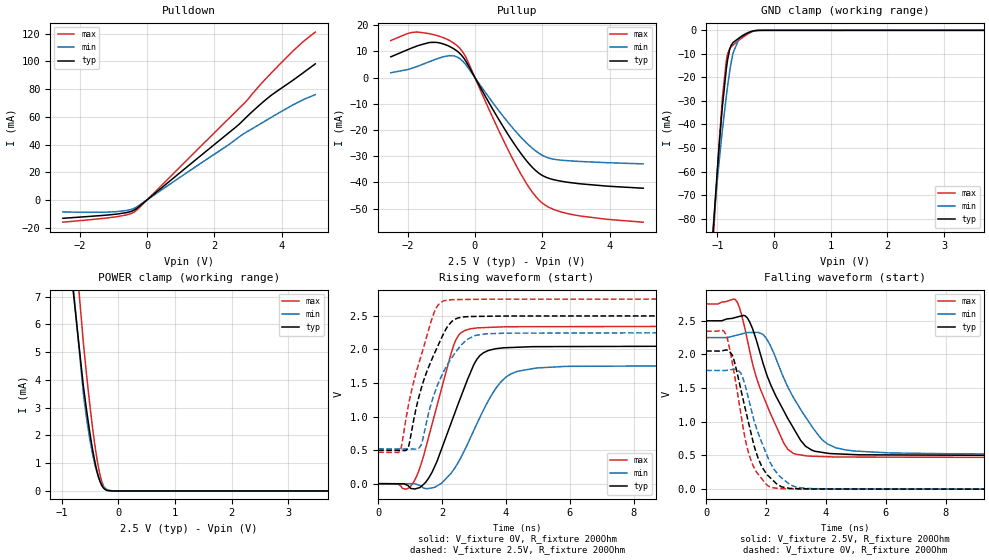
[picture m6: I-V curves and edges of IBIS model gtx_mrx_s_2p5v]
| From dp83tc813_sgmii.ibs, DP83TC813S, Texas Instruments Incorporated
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| gtx_mrx_s_2p5v
[Model]   gtx_mrx_s_2p5v
Model_type   I/O
Polarity   Non-Inverting
Enable   Active-Low
Vinl = 0.7
Vinh = 1.7
Vmeas = 1.25
Vref = 1.25
Cref = 2pF
Rref = 100000
|   typ   min   max
C_comp   2.76pF   2.73pF   2.77pF
[Voltage Range]   2.5   2.25   2.75
[Temperature Range]   27   150   -40
[Pullup Reference]   2.5   2.25   2.75
[Pulldown Reference]   0   0   0
[Power Clamp Reference]   2.5   2.25   2.75
[GND Clamp Reference]   0   0   0
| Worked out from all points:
|   slope of the pulldown table from 0 to 0.375 V, typ, clamps not added: 49.7 ohm
|   slope of the pullup table from 0 to 0.375 V, typ, clamps not added: 43.5 ohm
|   GND clamp passes 1 mA (typ) near -0.45 V on its own axis
|   POWER clamp passes 1 mA (typ) near -0.41 V on its own axis
|   falling waveform, V_fixture 2.5V, R_fixture 200Ohm: 20-80 % time 1.18ns typ, 1.28ns min, 1.01ns max; typ from 2.5 V to 0.498 V
|   rising waveform, V_fixture 0V, R_fixture 200Ohm: 20-80 % time 975ps typ, 1.12ns min, 794ps max; typ from 0 V to 2.05 V
|   rising waveform, V_fixture 2.5V, R_fixture 200Ohm: 20-80 % time 823ps typ, 856ps min, 727ps max; typ from 0.498 V to 2.5 V
|   falling waveform, V_fixture 0V, R_fixture 200Ohm: 20-80 % time 706ps typ, 814ps min, 592ps max; typ from 2.05 V to 0 V
[Pulldown]
|   Voltage   I(typ)   I(min)   I(max)
-2.5V     -13.29mA   -8.687mA   -16.1mA
-925mV    -10.31mA   -8.492mA   -12.22mA
-512.5mV  -8.603mA   -7.139mA   -10.18mA
-347.5mV  -6.835mA   -5.631mA   -8.211mA
2.638V    52.57mA    43.69mA    63.75mA
2.885V    58.13mA    47.96mA    69.7mA
3.462V    71.02mA    56.29mA    85.76mA
3.958V    80.11mA    63.41mA    98.27mA
4.633V    91.66mA    72.28mA    114.2mA
5V        98.27mA    76.01mA    121.2mA
[GND Clamp]
|   Voltage   I(typ)   I(min)   I(max)
-2.5V     -649.6mA   -557.1mA   -724.7mA
-1.097V   -92.84mA   -90.08mA   -98.6mA
-1.03V    -68.96mA   -71.19mA   -71.1mA
-962.5mV  -46.84mA   -53.94mA   -45.4mA
-917.5mV  -33.74mA   -43.48mA   -30.33mA
-835mV    -14.88mA   -26.4mA    -11.64mA
-782.5mV  -7.979mA   -17.25mA   -7.714mA
-722.5mV  -5.135mA   -9.451mA   -6.216mA
-617.5mV  -3.252mA   -3.474mA   -4.173mA
-497.5mV  -1.53mA    -1.353mA   -2.064mA
-265mV    -14.91uA   -36.81uA   -15.25uA
5V        0A         0A         0A
[Pullup]
|   Voltage   I(typ)   I(min)   I(max)
-2.5V     7.944mA    1.866mA    14.16mA
-1.847V   11.46mA    3.684mA    17.29mA
-1.315V   13.45mA    6.279mA    16.67mA
-752.5mV  11.89mA    8.383mA    14.16mA
-460mV    9.358mA    7.341mA    11.34mA
-257.5mV  5.988mA    4.704mA    7.488mA
642.5mV   -14.55mA   -11.48mA   -18.41mA
1.272V    -27.27mA   -21.43mA   -34.67mA
1.677V    -33.87mA   -26.64mA   -43.23mA
2.007V    -37.38mA   -29.68mA   -47.92mA
2.953V    -40.27mA   -31.87mA   -52.42mA
5V        -42.22mA   -32.93mA   -55.18mA
[POWER Clamp]
|   Voltage   I(typ)   I(min)   I(max)
-2.5V     111.4mA    76.2mA     154.9mA
-1.06V    12.26mA    13.09mA    16.05mA
-617.5mV  3.803mA    3.523mA    5.367mA
-557.5mV  2.879mA    2.591mA    4.147mA
-505mV    2.141mA    1.896mA    3.157mA
-445mV    1.398mA    1.242mA    2.137mA
-392.5mV  857.5uA    791.8uA    1.369mA
-347.5mV  495.5uA    495.4uA    828.3uA
-302.5mV  241.6uA    280.7uA    419.5uA
-220mV    36.63uA    73.03uA    55.79uA
-2.5mV    0A         70.01nA    0A
5V        0A         0A         0A
[Ramp]
R_load = 200
|   typ   min   max
dV/dt_r   1.23037/9.67486e-10   1.05666/1.12067e-09   1.40715/7.92973e-10
dV/dt_f   1.20096/1.16812e-09   1.03799/1.27155e-09   1.36848/1.00485e-09
[Falling Waveform]
V_fixture = 2.5V
V_fixture_min = 2.25V
V_fixture_max = 2.75V
R_fixture = 200Ohm
C_fixture = 0F
|   Time   V(typ)   V(min)   V(max)
0s        2.5V       2.25V      2.75V
1.029ns   2.555V     2.286V     2.785V
1.454ns   2.484V     2.325V     2.054V
1.924ns   1.839V     2.285V     1.366V
2.596ns   1.161V     1.649V     682.7mV
2.901ns   919.2mV    1.374V     534.6mV
3.324ns   636.6mV    1.07V      496.4mV
3.877ns   545.8mV    734.2mV    484.4mV
4.637ns   519.3mV    584.3mV    477.1mV
12ns      498.4mV    519.9mV    469.2mV
[Rising Waveform]
V_fixture = 0V
V_fixture_min = 0V
V_fixture_max = 0V
R_fixture = 200Ohm
C_fixture = 0F
|   Time   V(typ)   V(min)   V(max)
0s        25.62uV    133.3uV    11.85uV
855.4ps   -12.29mV   -959.5uV   -81.82mV
1.125ns   -77.92mV   -1.304mV   36.02mV
1.693ns   175mV      -62.08mV   895.2mV
2.363ns   1.004V     207.9mV    2.057V
2.722ns   1.456V     513.7mV    2.283V
3.298ns   1.95V      1.097V     2.325V
3.836ns   2.019V     1.511V     2.334V
4.377ns   2.032V     1.675V     2.338V
12ns      2.051V     1.761V     2.345V
[Rising Waveform]
V_fixture = 2.5V
V_fixture_min = 2.25V
V_fixture_max = 2.75V
R_fixture = 200Ohm
C_fixture = 0F
|   Time   V(typ)   V(min)   V(max)
0s        498.4mV    519.9mV    469.2mV
704.5ps   494.1mV    517mV      505.9mV
933.8ps   533.5mV    516mV      1.137V
1.347ns   1.416V     577.2mV    1.91V
1.762ns   1.94V      1.342V     2.561V
2.039ns   2.225V     1.66V      2.72V
2.314ns   2.42V      1.882V     2.74V
2.794ns   2.488V     2.149V     2.744V
3.401ns   2.494V     2.233V     2.748V
12ns      2.5V       2.25V      2.75V
[Falling Waveform]
|Gnd
V_fixture = 0V
V_fixture_min = 0V
V_fixture_max = 0V
R_fixture = 200Ohm
C_fixture = 0F
|   Time   V(typ)   V(min)   V(max)
0s        2.052V     1.763V     2.346V
599.3ps   2.061V     1.762V     2.342V
869.9ps   1.993V     1.777V     1.889V
1.154ns   1.494V     1.726V     1.138V
1.436ns   952.5mV    1.311V     511.8mV
1.748ns   446.7mV    823.1mV    216.9mV
2.124ns   177.7mV    409.7mV    34.5mV
2.751ns   15.09mV    84.29mV    5.592mV
3.37ns    4.468mV    10.49mV    1.985mV
12ns      25.7uV     133.3uV    11.98uV
